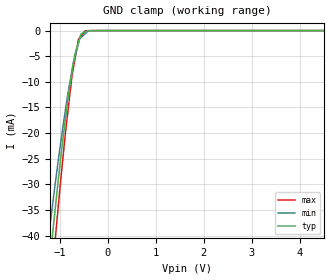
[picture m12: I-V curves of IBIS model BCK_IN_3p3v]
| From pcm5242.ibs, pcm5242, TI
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|   BCK_IN_3p3v
[Model]   BCK_IN_3p3v
Model_type   Input
Vinl = 0.99
Vinh = 2.31
|   typ   min   max
C_comp   1.426525397pF   1.374530485pF   1.444284221pF
[Voltage Range]   3.3   3   3.6
[Temperature Range]   27   105   -25
[Power Clamp Reference]   3.3   3   3.6
[GND Clamp Reference]   -0   -0   -0
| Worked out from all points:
|   GND clamp passes 1 mA (typ) near -0.57 V on its own axis
[GND Clamp]
|   Voltage   I(typ)   I(min)   I(max)
-3.3V     -526.5mA   -489.6mA   -552.8mA
-1.223V   -46.27mA   -39.34mA   -54.17mA
-1.139V   -38.52mA   -32.98mA   -45.18mA
-1.078V   -33.07mA   -28.51mA   -38.81mA
-882.5mV  -17.07mA   -15.34mA   -19.81mA
-746.7mV  -8.048mA   -7.686mA   -8.786mA
-689.8mV  -4.65mA    -5.27mA    -5.807mA
-610.8mV  -2.252mA   -2.464mA   -1.67mA
-557.7mV  -638.8uA   -1.348mA   -1.038mA
-475mV    -252.8uA   -630.3uA   -54.69uA
-230.4mV  -11.43uA   -497.9nA   -215.4nA
6.6V      0A         0A         0A
[POWER Clamp]
|   Voltage   I(typ)   I(min)   I(max)
-3.3V     0A         0A         0A
0V        0A         0A         0A
6.6V      0A         0A         0A
